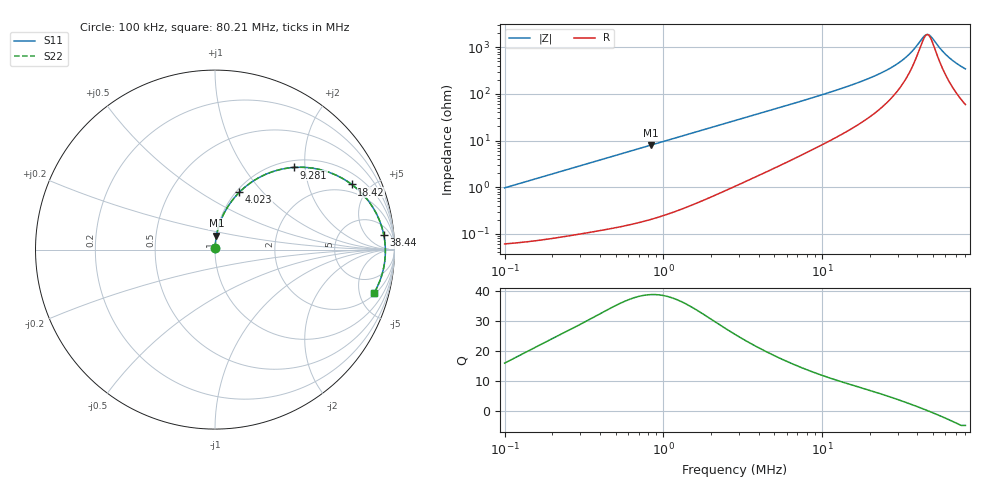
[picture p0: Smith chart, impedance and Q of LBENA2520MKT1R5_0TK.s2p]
! LBENA2520MKT1R5_0TK  S-PARAMETER MODEL  ( Standard Model )
! Model Generated by TAIYO YUDEN Corporation (http://www.ty-top.com)
! Version 1.0
! TAIYO YUDEN Control No. 20240828
! Copyright(c) 2024 TAIYO YUDEN CO.,LTD. All Rights Reserved.
! Product Description (link to TY-COMPAS)
! https://ds.yuden.co.jp/TYCOMPAS/or/detail?pn=LBENA2520MKT1R5M0TK&u=M
! Products Name : Inductors
! Characteristics :
!  Inductance : 1.5 [uH] , SRF(min) : - [Hz] , DC Resistance(max) : 0.057 [Ohm]
!  Rated Current : Saturation  3300 [mA] , Temp Rise  2800 [mA] (40 [degC])
!  Case Size : 2.5 x 2.0 / 0.098 x 0.079 [mm/inch] , Thickness : 1.2 / 0.047 [mm/inch]
!  (Conditions: Temperature = 25 [degC] , DC Bias Current = 0 [A])
! External Node Assignments :
!  1  o---GGG---o  2
! GND o---------o GND
! Frequency Range : 0.1MHz  -  80.209071MHz  [ 402 STEP ]
# MHz S RI R 50
! Freq[MHz].  S11 Real  S11 Imag  S21 Real  S21 Imag  S12 Real  S12 Imag  S22 Real  S22 Imag
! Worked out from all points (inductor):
!   401 points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, 100 kHz to 80.21 MHz, reference 50 ohm
!   read as one part in series: L = 1.53 uH near 103.4 kHz
!   highest Q = 38.8 at 835.8 kHz (marker M1), where L = 1.5 uH
!   self-resonance near 46.12 MHz
!   S11 on the Smith chart (normalised r, x): 100 kHz: 1.00, +0.02; 4.023 MHz: 1.04, +0.75; 9.281 MHz: 1.14, +1.76; 18.42 MHz: 1.53, +3.85; 38.44 MHz: 11, +16; 80.21 MHz: 2.18, -6.74
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0.1  0.000701 0.00963  0.9993 -0.00963  0.9993 -0.00963  0.000701 0.00963
0.306519  0.00186 0.0292  0.9981 -0.0292  0.9981 -0.0292  0.00186 0.0292
0.835778  0.0082 0.0782  0.9918 -0.0782  0.9918 -0.0782  0.0082 0.0782
0.939539  0.0101 0.0877  0.9899 -0.0877  0.9899 -0.0877  0.0101 0.0877
1.658723  0.0282 0.1511  0.9718 -0.1511  0.9718 -0.1511  0.0282 0.1511
2.832121  0.0742 0.2432  0.9258 -0.2432  0.9258 -0.2432  0.0742 0.2432
4.02331  0.1357 0.3194  0.8643 -0.3194  0.8643 -0.3194  0.1357 0.3194
5.811868  0.2416 0.3993  0.7584 -0.3993  0.7584 -0.3993  0.2416 0.3993
8.680988  0.4094 0.4547  0.5906 -0.4547  0.5906 -0.4547  0.4094 0.4547
9.281356  0.4414 0.4578  0.5586 -0.4578  0.5586 -0.4578  0.4414 0.4578
12.9665  0.6056 0.4403  0.3944 -0.4403  0.3944 -0.4403  0.6056 0.4403
18.4202  0.7618 0.3631  0.2382 -0.3631  0.2382 -0.3631  0.7618 0.3631
26.60888  0.8799 0.2345  0.1201 -0.2345  0.1201 -0.2345  0.8799 0.2345
32.52021  0.9203 0.1523  0.0797 -0.1523  0.0797 -0.1523  0.9203 0.1523
38.43783  0.9406 0.0804  0.0594 -0.0804  0.0594 -0.0804  0.9406 0.0804
43.93831  0.9483 0.0216  0.0517 -0.0216  0.0517 -0.0216  0.9483 0.0216
46.97704  0.9493 -0.00813  0.0507 0.00813  0.0507 0.00813  0.9493 -0.00813
49.39321  0.9488 -0.0305  0.0512 0.0305  0.0512 0.0305  0.9488 -0.0305
56.46141  0.942 -0.09  0.058 0.09  0.058 0.09  0.942 -0.09
62.41876  0.9317 -0.1345  0.0683 0.1345  0.0683 0.1345  0.9317 -0.1345
71.35092  0.9108 -0.193  0.0892 0.193  0.0892 0.193  0.9108 -0.193
80.20907  0.8855 -0.2428  0.1145 0.2428  0.1145 0.2428  0.8855 -0.2428
